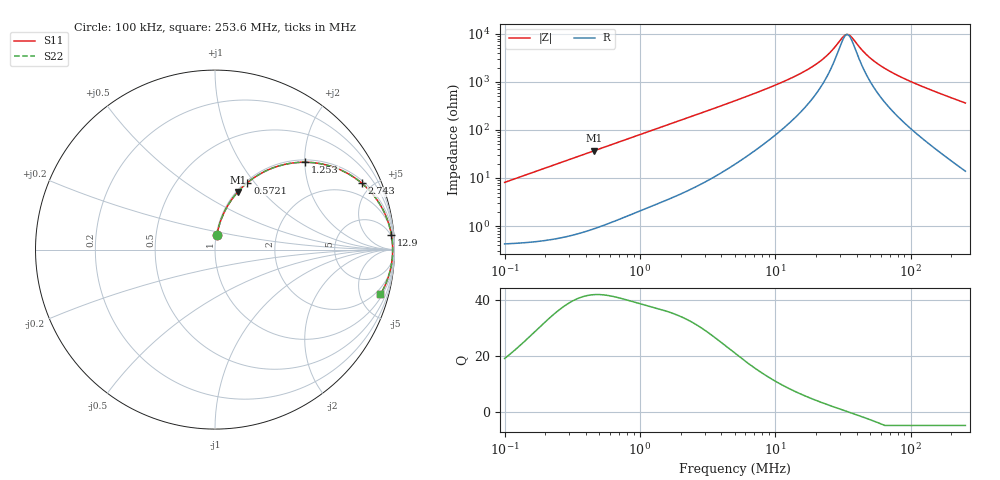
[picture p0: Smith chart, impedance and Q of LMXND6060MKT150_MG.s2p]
! LMXND6060MKT150_MG  S-PARAMETER MODEL  ( General Type )
! Model Generated by TAIYO YUDEN Corporation (https://www.yuden.co.jp/en/)
! Version 1.0
! TAIYO YUDEN Control No. 191025NI43SB-FBB
! Copyright(c) 2019 TAIYO YUDEN CO.,LTD. All Rights Reserved.
! Product Description (link to TY-COMPAS)
! https://ds.yuden.co.jp/TYCOMPAS/or/detail?pn=LMXND6060MKT150MMG&u=M
! Products Name : Inductors
! Characteristics :
!  Inductance : 15 uH , SRF(min) : 18 MHz , DC Resistance(max) : 0.354 Ohm
!  Rated Current : Saturation :800 mA , Temp Rise : 800 mA (40 degC)
!  Case Size : 6.0 x 6.0 / 0.236 x 0.236 [mm/inch] , Thickness : 1.2 / 0.047 [mm/inch]
!  (Conditions: Temperature = 25 degC , DC Bias Current/Voltage = 0A / 0V)
! External Node Assignments :
!  1  o---GGG---o  2
! GND o---------o GND
! Frequency Range : 0.1MHz  -  253.640152MHz  [ 402 STEP ]
# MHz S RI R 50
! Freq[MHz].  S11 Real  S11 Imag  S21 Real  S21 Imag  S12 Real  S12 Imag  S22 Real  S22 Imag
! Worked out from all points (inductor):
!   401 points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, 100 kHz to 253.6 MHz, reference 50 ohm
!   read as one part in series: L = 12.9 uH near 104 kHz
!   highest Q = 42.1 at 461.1 kHz (marker M1), where L = 12.8 uH
!   self-resonance near 33.7 MHz
!   S11 on the Smith chart (normalised r, x): 100 kHz: 1.01, +0.16; 572.1 kHz: 1.02, +0.92; 1.253 MHz: 1.05, +2.00; 2.743 MHz: 1.14, +4.37; 12.9 MHz: 4, +23; 253.6 MHz: 1.28, -7.29
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0.1  0.0107 0.0798  0.9893 -0.0798  0.9893 -0.0798  0.0107 0.0798
0.19855  0.0298 0.1551  0.9702 -0.1551  0.9702 -0.1551  0.0298 0.1551
0.371712  0.0881 0.2716  0.9119 -0.2716  0.9119 -0.2716  0.0881 0.2716
0.461129  0.1273 0.3216  0.8727 -0.3216  0.8727 -0.3216  0.1273 0.3216
0.572056  0.1808 0.3731  0.8192 -0.3731  0.8192 -0.3731  0.1808 0.3731
0.880381  0.3364 0.46  0.6636 -0.46  0.6636 -0.46  0.3364 0.46
1.252738  0.5002 0.4868  0.4998 -0.4868  0.4998 -0.4868  0.5002 0.4868
1.381698  0.5473 0.4844  0.4527 -0.4844  0.4527 -0.4844  0.5473 0.4844
2.004995  0.7126 0.4382  0.2874 -0.4382  0.2874 -0.4382  0.7126 0.4382
2.743356  0.819 0.369  0.181 -0.369  0.181 -0.369  0.819 0.369
5.03627  0.9333 0.2267  0.0667 -0.2267  0.0667 -0.2267  0.9333 0.2267
12.90076  0.9829 0.0817  0.0171 -0.0817  0.0171 -0.0817  0.9829 0.0817
18.72042  0.9876 0.046  0.0124 -0.046  0.0124 -0.046  0.9876 0.046
24.62993  0.9893 0.0239  0.0107 -0.0239  0.0107 -0.0239  0.9893 0.0239
31.77607  0.9898 0.00484  0.0102 -0.00484  0.0102 -0.00484  0.9898 0.00484
34.36706  0.9899 -0.0009  0.0101 0.0009  0.0101 0.0009  0.9899 -0.0009
36.44803  0.9898 -0.0052  0.0102 0.0052  0.0102 0.0052  0.9898 -0.0052
43.47794  0.9895 -0.0183  0.0105 0.0183  0.0105 0.0183  0.9895 -0.0183
49.87039  0.989 -0.0288  0.011 0.0288  0.011 0.0288  0.989 -0.0288
69.58603  0.9866 -0.0569  0.0134 0.0569  0.0134 0.0569  0.9866 -0.0569
120.4529  0.9756 -0.1177  0.0244 0.1177  0.0244 0.1177  0.9756 -0.1177
253.6402  0.9219 -0.2499  0.0781 0.2499  0.0781 0.2499  0.9219 -0.2499
